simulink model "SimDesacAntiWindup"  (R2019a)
settings: Solver=VariableStepAuto  StartTime=0.0  StopTime=16  RelTol=1e-5  AbsTol=1e-5
PreLoadFcn:
  | load ModeloTanqueLin
  | TanqueMezcladoLin.OutputDelay=[0.15;0];
  | s=tf('s');
  | Gact=1/(0.02*s+1);
libraries: cstblocks x6, simulink x4

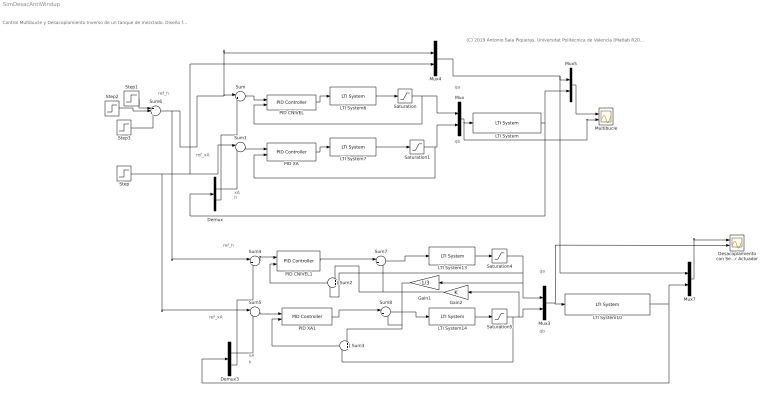
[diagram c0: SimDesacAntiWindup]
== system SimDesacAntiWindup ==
  note: (C) 2019 Antonio Sala Piqueras, Universitat Politecnica de Valencia [Matlab R2019a]
  note: Control Multibucle y Desacoplamiento Inverso de un tanque de mezclado. Diseño final con sensores de caudal + Antiwindup
  note: ref_xA
  note: ref_h
  note: h
  note: xA
  note: qb
  note: qa
  note: qa
  note: h
  note: ref_h
  note: ref_xA
  note: qb
  note: xA
  Demux : Demux  Outputs=2
  Demux3 : Demux  Outputs=2
  Desacoplamiento con Sensor Actuador : Scope  NumInputPorts=2
  Gain1 : Gain  Gain=-1/3
  Gain2 : Gain
  LTI System : cstblocks/LTI System  sys=TanqueMezcladoLin  IC=[]
  LTI System10 : cstblocks/LTI System  sys=TanqueMezcladoLin  IC=[]
  LTI System{6..7,13..14} (4 alike) : cstblocks/LTI System  sys=Gact  IC=[]
  Multibucle : Scope  NumInputPorts=2
  Mux{,3..5,7} (5 alike) : Mux  Inputs=2
  PID CNIVEL : simulink/Continuous/PID Controller  Controller=PID  Form=Parallel  TimeDomain=Continuous-time  SampleTime=-1  IntegratorMethod=Forward Euler  FilterMethod=Forward Euler  ControllerParametersSource=internal  P=3.5  I=6  D=0  UseFilter=on  N=100  TunerSelectOption=Transfer Function Based (PID Tuner App)  InitialConditionSource=internal  InitialConditionForIntegrator=0  InitialConditionForFilter=0  DifferentiatorICPrevScaledInput=0  ExternalReset=none  TrackingMode=on  Kt=1  LimitOutput=off  UpperSaturationLimit=inf  LowerSaturationLimit=-inf  LinearizeAsGain=on  AntiWindupMode=back-calculation  Kb=1  POutMin=[]  POutMax=[]  IOutMin=[]  IOutMax=[]  DOutMin=[]  DOutMax=[]  NOutMin=[]  NOutMax=[]  SumOutMin=[]  SumOutMax=[]  SaturationOutMin=[]  SaturationOutMax=[]  PParamMin=[]  PParamMax=[]  IParamMin=[]  IParamMax=[]  DParamMin=[]  DParamMax=[]  NParamMin=[]  NParamMax=[]  KbParamMin=[]  KbParamMax=[]  KtParamMin=[]  KtParamMax=[]  KbOutMin=[]  KbOutMax=[]  KtOutMin=[]  KtOutMax=[]  IntegratorOutMin=[]  IntegratorOutMax=[]  FilterOutMin=[]  FilterOutMax=[]  SumI1OutMin=[]  SumI1OutMax=[]  SumI2OutMin=[]  SumI2OutMax=[]  SumI3OutMin=[]  SumI3OutMax=[]  SumI4OutMin=[]  SumI4OutMax=[]  SumDOutMin=[]  SumDOutMax=[]  DifferentiatorOutMin=[]  DifferentiatorOutMax=[]  FilterDiffOutCoefMin=[]  FilterDiffOutCoefMax=[]  ReciprocalOutMin=[]  ReciprocalOutMax=[]  SumDenOutMin=[]  SumDenOutMax=[]  SumNumOutMin=[]  SumNumOutMax=[]  DivideOutMin=[]  DivideOutMax=[]  IntegratorContinuousStateAttributes=''  IntegratorStateMustResolveToSignalObject=off  IntegratorRTWStateStorageClass=Auto  FilterContinuousStateAttributes=''  FilterStateMustResolveToSignalObject=off  FilterRTWStateStorageClass=Auto  ParallelPVariant=InternalParameters  IdealPVariant=Disabled  IVariant=InternalParameters  DVariant=InternalParameters  IntegratorVariant=Continuous  SatVariant=Disabled  AWVariant=Passthrough  PCopyVariant=Disabled  TRVariant=Enabled  FdbkBlocksVariant=Forward  IdealPFdbkVariant=Disabled  SatFdbkVariant=Disabled  DerivativeFilterVariant=ContFilter  NVariant=InternalParameters  NCopyVariant=Disabled  FilterICVariant=InternalICsFilter  IntegratorICVariant=InternalICs  ExternalResetVariant=Disabled  TRSumVariant=TrackingMode  SumFdbkVariant=Disabled  SumVariant=Sum_PID
  PID CNIVEL1 : simulink/Continuous/PID Controller  Controller=PID  Form=Parallel  TimeDomain=Continuous-time  SampleTime=-1  IntegratorMethod=Forward Euler  FilterMethod=Forward Euler  ControllerParametersSource=internal  P=3.5  I=6  D=0  UseFilter=on  N=100  TunerSelectOption=Transfer Function Based (PID Tuner App)  InitialConditionSource=internal  InitialConditionForIntegrator=0  InitialConditionForFilter=0  DifferentiatorICPrevScaledInput=0  ExternalReset=none  TrackingMode=on  Kt=1  LimitOutput=off  UpperSaturationLimit=inf  LowerSaturationLimit=-inf  LinearizeAsGain=on  AntiWindupMode=back-calculation  Kb=1  POutMin=[]  POutMax=[]  IOutMin=[]  IOutMax=[]  DOutMin=[]  DOutMax=[]  NOutMin=[]  NOutMax=[]  SumOutMin=[]  SumOutMax=[]  SaturationOutMin=[]  SaturationOutMax=[]  PParamMin=[]  PParamMax=[]  IParamMin=[]  IParamMax=[]  DParamMin=[]  DParamMax=[]  NParamMin=[]  NParamMax=[]  KbParamMin=[]  KbParamMax=[]  KtParamMin=[]  KtParamMax=[]  KbOutMin=[]  KbOutMax=[]  KtOutMin=[]  KtOutMax=[]  IntegratorOutMin=[]  IntegratorOutMax=[]  FilterOutMin=[]  FilterOutMax=[]  SumI1OutMin=[]  SumI1OutMax=[]  SumI2OutMin=[]  SumI2OutMax=[]  SumI3OutMin=[]  SumI3OutMax=[]  SumI4OutMin=[]  SumI4OutMax=[]  SumDOutMin=[]  SumDOutMax=[]  DifferentiatorOutMin=[]  DifferentiatorOutMax=[]  FilterDiffOutCoefMin=[]  FilterDiffOutCoefMax=[]  ReciprocalOutMin=[]  ReciprocalOutMax=[]  SumDenOutMin=[]  SumDenOutMax=[]  SumNumOutMin=[]  SumNumOutMax=[]  DivideOutMin=[]  DivideOutMax=[]  IntegratorContinuousStateAttributes=''  IntegratorStateMustResolveToSignalObject=off  IntegratorRTWStateStorageClass=Auto  FilterContinuousStateAttributes=''  FilterStateMustResolveToSignalObject=off  FilterRTWStateStorageClass=Auto  ParallelPVariant=InternalParameters  IdealPVariant=Disabled  IVariant=InternalParameters  DVariant=InternalParameters  IntegratorVariant=Continuous  SatVariant=Disabled  AWVariant=Passthrough  PCopyVariant=Disabled  TRVariant=Enabled  FdbkBlocksVariant=Forward  IdealPFdbkVariant=Disabled  SatFdbkVariant=Disabled  DerivativeFilterVariant=ContFilter  NVariant=InternalParameters  NCopyVariant=Disabled  FilterICVariant=InternalICsFilter  IntegratorICVariant=InternalICs  ExternalResetVariant=Disabled  TRSumVariant=TrackingMode  SumFdbkVariant=Disabled  SumVariant=Sum_PID
  PID XA : simulink/Continuous/PID Controller  Controller=PID  Form=Parallel  TimeDomain=Continuous-time  SampleTime=-1  IntegratorMethod=Forward Euler  FilterMethod=Forward Euler  ControllerParametersSource=internal  P=3.75  I=12  D=0  UseFilter=on  N=100  TunerSelectOption=Transfer Function Based (PID Tuner App)  InitialConditionSource=internal  InitialConditionForIntegrator=0  InitialConditionForFilter=0  DifferentiatorICPrevScaledInput=0  ExternalReset=none  TrackingMode=on  Kt=1  LimitOutput=off  UpperSaturationLimit=inf  LowerSaturationLimit=-inf  LinearizeAsGain=on  AntiWindupMode=back-calculation  Kb=1  POutMin=[]  POutMax=[]  IOutMin=[]  IOutMax=[]  DOutMin=[]  DOutMax=[]  NOutMin=[]  NOutMax=[]  SumOutMin=[]  SumOutMax=[]  SaturationOutMin=[]  SaturationOutMax=[]  PParamMin=[]  PParamMax=[]  IParamMin=[]  IParamMax=[]  DParamMin=[]  DParamMax=[]  NParamMin=[]  NParamMax=[]  KbParamMin=[]  KbParamMax=[]  KtParamMin=[]  KtParamMax=[]  KbOutMin=[]  KbOutMax=[]  KtOutMin=[]  KtOutMax=[]  IntegratorOutMin=[]  IntegratorOutMax=[]  FilterOutMin=[]  FilterOutMax=[]  SumI1OutMin=[]  SumI1OutMax=[]  SumI2OutMin=[]  SumI2OutMax=[]  SumI3OutMin=[]  SumI3OutMax=[]  SumI4OutMin=[]  SumI4OutMax=[]  SumDOutMin=[]  SumDOutMax=[]  DifferentiatorOutMin=[]  DifferentiatorOutMax=[]  FilterDiffOutCoefMin=[]  FilterDiffOutCoefMax=[]  ReciprocalOutMin=[]  ReciprocalOutMax=[]  SumDenOutMin=[]  SumDenOutMax=[]  SumNumOutMin=[]  SumNumOutMax=[]  DivideOutMin=[]  DivideOutMax=[]  IntegratorContinuousStateAttributes=''  IntegratorStateMustResolveToSignalObject=off  IntegratorRTWStateStorageClass=Auto  FilterContinuousStateAttributes=''  FilterStateMustResolveToSignalObject=off  FilterRTWStateStorageClass=Auto  ParallelPVariant=InternalParameters  IdealPVariant=Disabled  IVariant=InternalParameters  DVariant=InternalParameters  IntegratorVariant=Continuous  SatVariant=Disabled  AWVariant=Passthrough  PCopyVariant=Disabled  TRVariant=Enabled  FdbkBlocksVariant=Forward  IdealPFdbkVariant=Disabled  SatFdbkVariant=Disabled  DerivativeFilterVariant=ContFilter  NVariant=InternalParameters  NCopyVariant=Disabled  FilterICVariant=InternalICsFilter  IntegratorICVariant=InternalICs  ExternalResetVariant=Disabled  TRSumVariant=TrackingMode  SumFdbkVariant=Disabled  SumVariant=Sum_PID
  PID XA1 : simulink/Continuous/PID Controller  Controller=PID  Form=Parallel  TimeDomain=Continuous-time  SampleTime=-1  IntegratorMethod=Forward Euler  FilterMethod=Forward Euler  ControllerParametersSource=internal  P=3.75  I=12  D=0  UseFilter=on  N=100  TunerSelectOption=Transfer Function Based (PID Tuner App)  InitialConditionSource=internal  InitialConditionForIntegrator=0  InitialConditionForFilter=0  DifferentiatorICPrevScaledInput=0  ExternalReset=none  TrackingMode=on  Kt=1  LimitOutput=off  UpperSaturationLimit=inf  LowerSaturationLimit=-inf  LinearizeAsGain=on  AntiWindupMode=back-calculation  Kb=1  POutMin=[]  POutMax=[]  IOutMin=[]  IOutMax=[]  DOutMin=[]  DOutMax=[]  NOutMin=[]  NOutMax=[]  SumOutMin=[]  SumOutMax=[]  SaturationOutMin=[]  SaturationOutMax=[]  PParamMin=[]  PParamMax=[]  IParamMin=[]  IParamMax=[]  DParamMin=[]  DParamMax=[]  NParamMin=[]  NParamMax=[]  KbParamMin=[]  KbParamMax=[]  KtParamMin=[]  KtParamMax=[]  KbOutMin=[]  KbOutMax=[]  KtOutMin=[]  KtOutMax=[]  IntegratorOutMin=[]  IntegratorOutMax=[]  FilterOutMin=[]  FilterOutMax=[]  SumI1OutMin=[]  SumI1OutMax=[]  SumI2OutMin=[]  SumI2OutMax=[]  SumI3OutMin=[]  SumI3OutMax=[]  SumI4OutMin=[]  SumI4OutMax=[]  SumDOutMin=[]  SumDOutMax=[]  DifferentiatorOutMin=[]  DifferentiatorOutMax=[]  FilterDiffOutCoefMin=[]  FilterDiffOutCoefMax=[]  ReciprocalOutMin=[]  ReciprocalOutMax=[]  SumDenOutMin=[]  SumDenOutMax=[]  SumNumOutMin=[]  SumNumOutMax=[]  DivideOutMin=[]  DivideOutMax=[]  IntegratorContinuousStateAttributes=''  IntegratorStateMustResolveToSignalObject=off  IntegratorRTWStateStorageClass=Auto  FilterContinuousStateAttributes=''  FilterStateMustResolveToSignalObject=off  FilterRTWStateStorageClass=Auto  ParallelPVariant=InternalParameters  IdealPVariant=Disabled  IVariant=InternalParameters  DVariant=InternalParameters  IntegratorVariant=Continuous  SatVariant=Disabled  AWVariant=Passthrough  PCopyVariant=Disabled  TRVariant=Enabled  FdbkBlocksVariant=Forward  IdealPFdbkVariant=Disabled  SatFdbkVariant=Disabled  DerivativeFilterVariant=ContFilter  NVariant=InternalParameters  NCopyVariant=Disabled  FilterICVariant=InternalICsFilter  IntegratorICVariant=InternalICs  ExternalResetVariant=Disabled  TRSumVariant=TrackingMode  SumFdbkVariant=Disabled  SumVariant=Sum_PID
  Saturation{,1,4..5} (4 alike) : Saturate  UpperLimit=2  LowerLimit=-2
  Step : Step  After=.2  SampleTime=0
  Step1 : Step  Time=4  After=0.4  SampleTime=0
  Step2 : Step  Time=7.5  After=1.25  SampleTime=0
  Step3 : Step  Time=11  After=-1.65  SampleTime=0
  Sum{,4,7..8} (4 alike) : Sum  Inputs=|+-
  Sum1 : Sum  Inputs=|-+
  Sum2 : Sum
  Sum3 : Sum
  Sum5 : Sum  Inputs=|-+
  Sum6 : Sum  Inputs=+++
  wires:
  LTI System/1 -> Demux/1, Mux5/2
  Mux/1 -> Multibucle/2, LTI System/1
  Sum/1 -> PID CNIVEL/1
  PID XA/1 -> LTI System7/1
  Demux/2 -> Sum/2
  Demux/1 -> Sum1/2
  PID CNIVEL/1 -> LTI System6/1
  Sum1/1 -> PID XA/1
  Demux3/2 -> Sum4/2
  Mux3/1 -> Desacoplamiento con Sensor Actuador/2, LTI System10/1
  Demux3/1 -> Sum5/2
  Sum6/1 -> Sum4/1, Mux4/1, Sum/1
  Sum4/1 -> PID CNIVEL1/1
  Sum5/1 -> PID XA1/1
  LTI System10/1 -> Mux7/2, Demux3/1
  Step1/1 -> Sum6/1
  Step2/1 -> Sum6/2
  PID CNIVEL1/1 -> Sum7/1
  PID XA1/1 -> Sum8/1
  Sum7/1 -> LTI System13/1
  Sum8/1 -> LTI System14/1
  Gain1/1 -> Sum3/1, Sum8/2
  Gain2/1 -> Sum2/1, Sum7/2
  LTI System6/1 -> Saturation/1
  Saturation/1 -> PID CNIVEL/2, Mux/1
  LTI System7/1 -> Saturation1/1
  Saturation1/1 -> PID XA/2, Mux/2
  LTI System13/1 -> Saturation4/1
  Saturation4/1 -> Sum2/2, Gain1/1, Mux3/1
  LTI System14/1 -> Saturation5/1
  Saturation5/1 -> Sum3/2, Gain2/1, Mux3/2
  Mux4/1 -> Mux7/1, Mux5/1
  Mux5/1 -> Multibucle/1
  Mux7/1 -> Desacoplamiento con Sensor Actuador/1
  Step/1 -> Sum5/1, Mux4/2, Sum1/1
  Step3/1 -> Sum6/3
  Sum2/1 -> PID CNIVEL1/2
  Sum3/1 -> PID XA1/2
